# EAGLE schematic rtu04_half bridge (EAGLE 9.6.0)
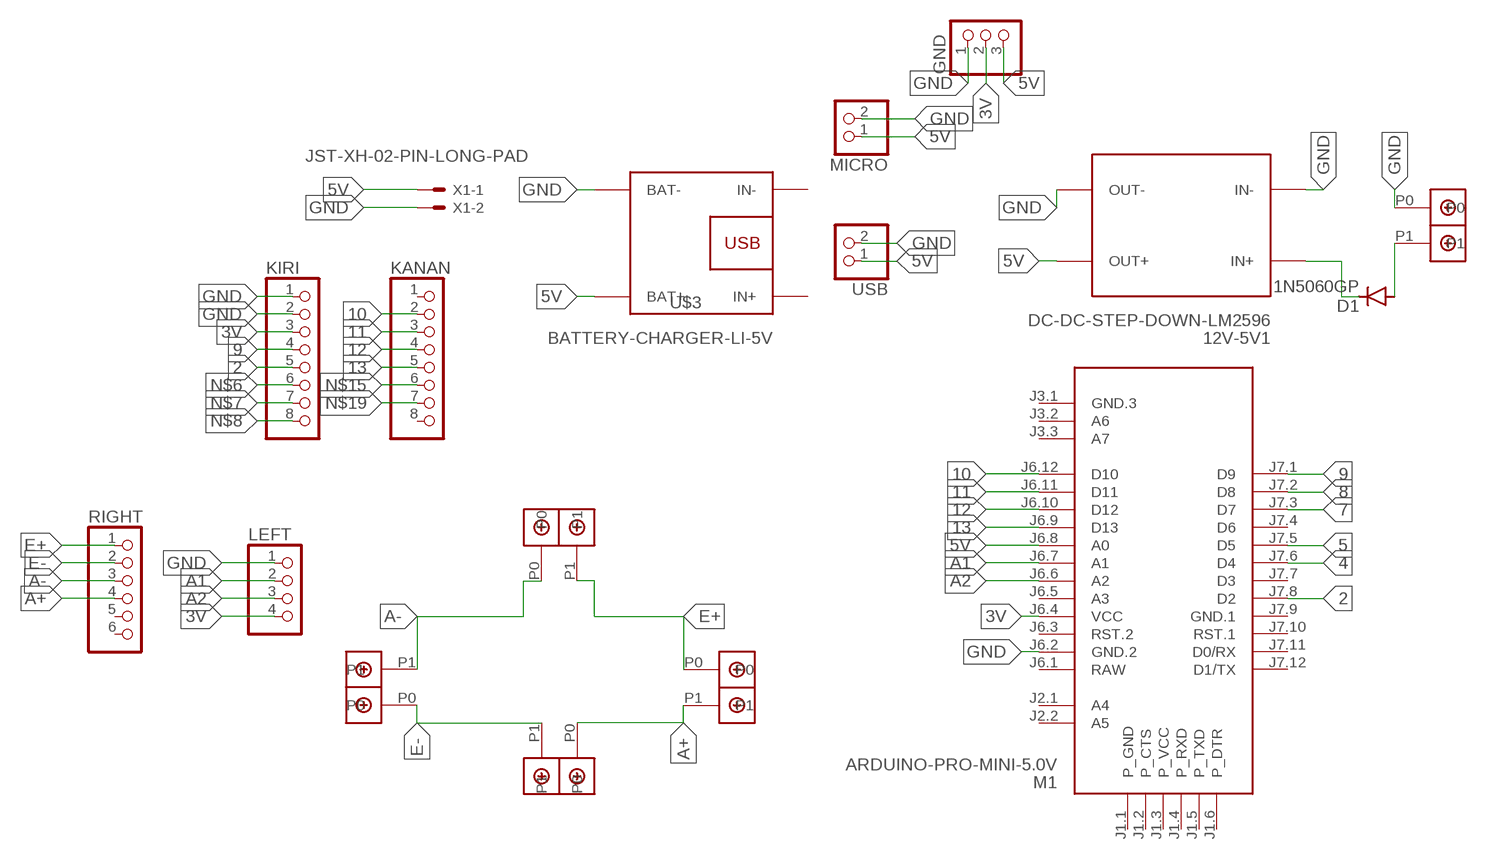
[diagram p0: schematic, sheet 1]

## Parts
12V-5V1  DC-DC-STEP-DOWN-LM2596  [DC-DC-STEP-DOWN-LM2596]
D1  1N5060GP  [DO15-12]
GND  PINHD-1X3  [1X03]
KANAN  PINHD-1X8  [1X08]
KIRI  PINHD-1X8  [1X08]
LEFT  PINHD-1X4  [1X04]
M1  ARDUINO-PRO-MINI-5.0V  [ARDUINO-PRO-MINI]
MICRO  PINHD-1X2  [1X02]
RIGHT  PINHD-1X6  [1X06]
U$1  DBCONN-1X2  [DBCONN-1X2]
U$2  DBCONN-1X2  [DBCONN-1X2]
U$3  BATTERY-CHARGER-LI-5V  [BATTERY-CHARGER-LI-5V]
U$4  DBCONN-1X2  [DBCONN-1X2]
U$5  DBCONN-1X2  [DBCONN-1X2]
U$6  DBCONN-1X2  [DBCONN-1X2]
USB  PINHD-1X2  [1X02]
X1  JST-XH-02-PIN-LONG-PAD  [JST-XH-02-PACKAGE-LONG-PAD]

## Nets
2: KIRI.5 M1.J7.8(D2)
3V: GND.2 KIRI.3 LEFT.4 M1.J6.4(VCC)
4: M1.J7.6(D4)
5: M1.J7.5(D5)
5V: 12V-5V1.OUT+ GND.3 M1.J6.8(A0) MICRO.1 U$3.BAT+ USB.1 X1.1
7: M1.J7.3(D7)
8: M1.J7.2(D8)
9: KIRI.4 M1.J7.1(D9)
10: KANAN.2 M1.J6.12(D10)
11: KANAN.3 M1.J6.11(D11)
12: KANAN.4 M1.J6.10(D12)
13: KANAN.5 M1.J6.9(D13)
A1: LEFT.2 M1.J6.7(A1)
A2: LEFT.3 M1.J6.6(A2)
A+: RIGHT.4 U$2.P0 U$4.P1
A-: RIGHT.3 U$5.P0 U$6.P1
E+: RIGHT.1 U$4.P0 U$5.P1
E-: RIGHT.2 U$2.P1 U$6.P0
GND: 12V-5V1.IN- 12V-5V1.OUT- GND.1 KIRI.1 KIRI.2 LEFT.1 M1.J6.2(GND.2) MICRO.2 U$1.P0 U$3.BAT- USB.2 X1.2
N$1: 12V-5V1.IN+ D1.C
N$2: D1.A U$1.P1
N$6: KIRI.6
N$7: KIRI.7
N$8: KIRI.8
N$15: KANAN.6
N$19: KANAN.7
Unconnected: KANAN.1 KANAN.8 M1.J1.1(P_GND) M1.J1.2(P_CTS) M1.J1.3(P_VCC) M1.J1.4(P_RXD) M1.J1.5(P_TXD) M1.J1.6(P_DTR) M1.J2.1(A4) M1.J2.2(A5) M1.J3.1(GND.3) M1.J3.2(A6) M1.J3.3(A7) M1.J6.3(RST.2) M1.J6.5(A3) M1.J7.4(D6) M1.J7.7(D3) M1.J7.10(RST.1) M1.J7.11(D0/RX) M1.J7.12(D1/TX) RIGHT.5 RIGHT.6 U$3.IN+ U$3.IN-

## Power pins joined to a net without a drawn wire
GND.1: M1.J7.9(GND.1)
RAW: M1.J6.1(RAW)

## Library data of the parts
12V-5V1 = diy-modules:DC-DC-STEP-DOWN-LM2596: DC/DC Step-Down Regulator based on LM2596-ADJ chip LM2596 datasheet available here: http://www.ti.com/lit/ds/symlink/lm2596.pdf Click here to find device on ebay.com
D1 = diode:1N5060GP: DIODE
GND = pinhead:PINHD-1X3: PIN HEADER
KANAN KIRI = pinhead:PINHD-1X8: PIN HEADER
LEFT = pinhead:PINHD-1X4: PIN HEADER
M1 = diy-modules:ARDUINO-PRO-MINI-*: Arduino Pro Mini and compatible devices More details available here: https://www.arduino.cc/en/Main/ArduinoBoardProMini Click here to find device on ebay.com
MICRO USB = pinhead:PINHD-1X2: PIN HEADER
RIGHT = pinhead:PINHD-1X6: PIN HEADER
U$1 U$2 U$4-U$6 = Terminal Block Connector:DBCONN-1X2
U$3 = diy-modules (1):BATTERY-CHARGER-LI-5V: Lithium Battery 5V Charger More details available here: http://www.buildcircuit.com/how-to-use-micro-usb-5v-1a-lithium-battery-charging-board-charger-module/ Click here to find device on ebay.com
X1 = Rembrandt Electronics - JST XH Connectors v1-0:JST-XH-02-PIN: JST XH Connector 2 Pin

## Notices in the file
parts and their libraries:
diy-modules: Released under the Creative Commons Attribution 4.0 International License: http://creativecommons.org/licenses/by/4.0
